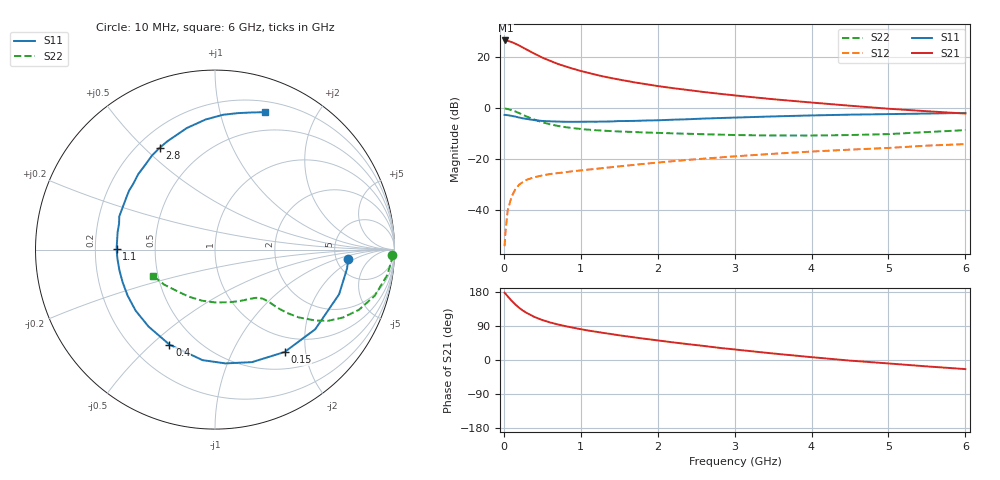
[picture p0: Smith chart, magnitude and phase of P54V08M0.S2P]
! SIEMENS Small Signal Semiconductors
! BFP183
! Si NPN RF Bipolar Junction Transistor in SOT143
! VCE = 4 V  IC = 8 mA
! Common Emitter S-Parameters:  March  1996
# GHz  S  MA  R  50
!  f  S11  S21  S12  S22
! GHz  MAG  ANG  MAG  ANG  MAG  ANG  MAG  ANG
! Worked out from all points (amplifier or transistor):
!   36 points, 10 MHz to 6 GHz, reference 50 ohm
!   highest |S21| = 26.6 dB at 20 MHz (marker M1)
!   |S21| within 3 dB of that: start of sweep to 261 MHz
!   unconditionally stable (mu >= 1): 1.292 GHz to 5.627 GHz
!   at 250 MHz: K = 0.28, MSG = 26.3 dB, |S12| = -28.8 dB
!   at 1.4 GHz: K = 1.04, MAG = 16.3 dB, |S12| = -23.0 dB
!   at 6 GHz: K = 0.94, MSG = 6.0 dB, |S12| = -14.0 dB
!   lowest NFmin = 1.30 dB at 450 MHz
!   S11 on the Smith chart (normalised r, x): 10 MHz: 6.46, -1.50; 150 MHz: 0.75, -1.63; 400 MHz: 0.35, -0.57; 1.1 GHz: 0.29, +0.00; 2.8 GHz: 0.29, +0.56; 6 GHz: 0.30, +1.38
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0.01  0.744 -4.0  21.35 177.5  0.002 86.9  0.989 -1.7
0.02  0.7433 -8.1  21.37 175.4  0.0036 84.1  0.9858 -3.3
0.05  0.7349 -19.8  20.96 167.9  0.01 82.6  0.9711 -8.3
0.1  0.7133 -38.5  19.9 156.7  0.0185 70.5  0.9265 -16.1
0.15  0.6899 -55.8  18.46 146.5  0.0261 63.8  0.8693 -22.7
0.2  0.66 -71.8  17.02 137.6  0.0321 58.4  0.8065 -28.0
0.25  0.6366 -84.8  15.43 130.0  0.0363 52.9  0.7446 -32.2
0.3  0.6198 -96.4  14.1 123.9  0.0401 49.7  0.6879 -35.1
0.4  0.5871 -115.6  11.72 113.4  0.0449 44.2  0.6004 -39.0
0.5  0.5665 -130.8  9.861 105.5  0.0485 40.9  0.535 -41.3
0.6  0.5579 -142.4  8.562 99.2  0.0517 39.8  0.4874 -42.6
0.7  0.5504 -152.1  7.426 93.9  0.0539 38.8  0.4532 -43.4
0.9  0.5449 -167.7  5.966 85.3  0.0589 38.3  0.41 -44.5
1.1  0.5484 179.7  4.949 77.6  0.0632 38.5  0.3822 -45.8
1.5  0.5644 160.9  3.66 65.1  0.0731 39.7  0.3524 -49.7
1.8  0.5744 148.7  3.055 56.8  0.0813 39.8  0.3384 -53.9
2.2  0.5996 135.5  2.487 46.5  0.0924 39.3  0.3242 -60.5
2.8  0.6455 118.6  1.934 32.1  0.1091 37.2  0.3058 -72.8
3.5  0.6951 103.1  1.511 17.2  0.1288 33.9  0.2944 -90.0
4.5  0.7528 86.5  1.126 -1.6  0.1555 27.4  0.3001 -119.3
5.5  0.791 75.0  0.879 -16.9  0.186 21.3  0.3433 -145.2
6  0.8143 70.1  0.79 -24.0  0.1997 17.0  0.3743 -156.9
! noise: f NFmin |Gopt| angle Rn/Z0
0.45  1.3  0.17  43  0.21
0.9  1.35  0.21  115  0.2
1.8  2.05  0.33  -177  0.14
